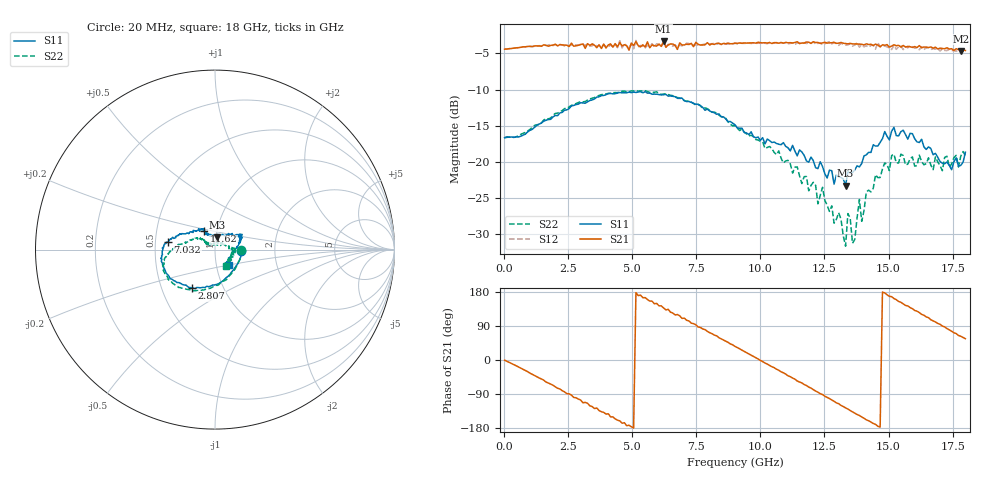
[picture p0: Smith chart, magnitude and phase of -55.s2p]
!Agilent Technologies,N5230A,US43500223,A.07.50.48
!Agilent N5230A: A.07.50.48
!Date: Saturday, January 16, 2016 19:59:59
!Correction: S11(Full 2 Port(1,2))
!S21(Full 2 Port(1,2))
!S12(Full 2 Port(1,2))
!S22(Full 2 Port(1,2))
!S2P File: Measurements: S11, S21, S12, S22:
# Hz S  dB  R 50
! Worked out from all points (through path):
!   201 points, 20 MHz to 18 GHz, reference 50 ohm
!   highest |S21| = -3.27 dB at 6.223 GHz (marker M1); lowest = -4.6 dB at 17.82 GHz (marker M2)
!   group delay of S21, straight-line fit = 103 ps
!   lowest |S11| = -23.2 dB at 13.33 GHz (marker M3), VSWR 1.15, Z = 50.6 + j6.91 ohm
!   |S11| at or under -10 dB: start of sweep to end of sweep
!   |S22| runs from -31.6 to -10.1 dB; largest |S21 - S12| = 0.09
!   S11 on the Smith chart (normalised r, x): 20 MHz: 1.35, -0.02; 2.807 GHz: 0.71, -0.32; 7.032 GHz: 0.58, +0.05; 11.62 GHz: 0.87, +0.18; 18 GHz: 1.15, -0.20
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2e7  -16.63 -2.2  -4.40 -0.5  -4.41 -0.6  -16.63 -1.9
1.2786e9  -14.92 -75.3  -3.95 -44.3  -3.96 -44.2  -14.84 -72.6
2.8069e9  -12.06 -121.4  -3.94 -99.7  -3.81 -101.3  -11.93 -115.2
3.0766e9  -11.83 -127.1  -3.68 -112.8  -3.72 -112.1  -11.69 -120.7
4.515e9  -10.39 -154.8  -3.49 -160.5  -3.23 -162.6  -10.25 -145.5
6.0433e9  -10.67 -178.9  -3.69 143.0  -3.86 138.8  -10.54 -163.7
6.2231e9  -10.70 177.7  -3.27 137.3  -3.57 134.9  -10.61 -166.7
7.0322e9  -11.52 170.6  -3.82 110.4  -3.80 106.8  -11.51 -174.1
9.01e9  -14.86 149.0  -3.56 35.9  -3.60 32.3  -14.98 169.3
1.03585e10  -17.03 126.8  -3.48 -14.4  -3.54 -18.1  -17.86 150.6
1.16171e10  -18.60 120.2  -3.55 -60.3  -3.59 -64.7  -22.97 142.5
1.20666e10  -19.82 115.4  -3.38 -78.2  -3.40 -82.8  -22.80 140.9
1.33252e10  -23.25 81.3  -3.62 -126.4  -3.83 -131.2  -31.63 105.3
1.34151e10  -21.34 80.6  -3.67 -129.5  -3.81 -134.3  -27.12 91.0
1.35949e10  -21.45 68.0  -3.68 -136.8  -3.97 -143.0  -31.22 68.8
1.38646e10  -20.68 56.8  -3.70 -146.4  -4.13 -152.5  -25.18 42.6
1.39545e10  -20.20 54.6  -3.73 -150.4  -3.77 -154.8  -28.19 35.7
1.44939e10  -17.80 41.4  -3.70 -169.9  -4.38 -173.7  -21.75 13.2
1.50333e10  -16.95 31.8  -4.11 167.9  -4.26 162.1  -21.19 4.6
1.65616e10  -17.90 5.7  -4.18 111.7  -4.21 104.1  -19.42 -27.7
1.78202e10  -20.46 -47.2  -4.64 62.6  -4.91 55.4  -19.18 -47.7
1.8e10  -18.65 -48.5  -4.58 56.2  -4.72 47.7  -19.15 -57.2
